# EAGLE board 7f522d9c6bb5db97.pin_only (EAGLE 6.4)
REV: B

Size 25.4 x 25.4 mm. Coordinates in mm from the lower left corner, seen from the top.
Outline: circle at 12.7,12.7 radius 12.7
Copper layers (1*16): Top 0.035mm / dielectric 1.5mm / Bottom 0.035mm
Design rules "adafruit *": minimum track width 8mil, minimum drill 15.5mil, track to track 8mil, track to pad 8mil, pad to pad 8mil, via to via 8mil, smd to smd 8mil, copper to edge 10mil, drill to drill 8mil, minimum pad ring 10mil, minimum via ring 8mil, stop-mask expansion 4mil, vias tented up to drill 20mil, thermal gap 10mil
Net classes: 1 GND: width 0.305 mm; 2 VIN: width 0.305 mm; 3 +3.3: width 0.305 mm
Holes 2.8 mm at 2.54,12.7 22.86,12.7

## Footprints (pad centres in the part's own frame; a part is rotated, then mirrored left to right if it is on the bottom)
0805-NO = smd 1.24 x 1.5: 1 -0.95,0; 2 0.95,0
FIDUCIAL_1MM = smd 1 x 1: 1 0,0
SEWALLI = drill 3.2: P$1 0,0.508
SOT363 = smd 0.5 x 0.5: 1 -0.75,-0.9; 3 0.75,-0.9; 4 0.75,0.9; 6 -0.75,0.9 | smd 0.4 x 0.5: 2 0,-0.9; 5 0,0.9
RESPACK_4X0603 = smd 0.45 x 0.9: 1 -1.3,-0.85; 2 -0.4,-0.85; 3 0.4,-0.85; 4 1.3,-0.85; 5 1.3,0.85; 6 0.4,0.85; 7 -0.4,0.85; 8 -1.3,0.85
SOLDERJUMPER_2WAY_OPEN_NOPASTE = smd 1.168 x 1.6: 1 -1.397,0; 2 0,0; 3 1.397,0
SOT23-5 = smd 0.55 x 1.2: 1 -0.95,-1.3; 2 0,-1.3; 3 0.95,-1.3; 4 0.95,1.3; 5 -0.95,1.3
TSL2561_FN = smd 1.3 x 0.4: ADR -0.8,0; CLK 0.8,-0.65; DATA 0.8,0.65; INT 0.8,0; VDD -0.8,0.65; VSS -0.8,-0.65
JSTPH4 = smd 1 x 4.6: 1 -3,-3.7; 2 -1,-3.7; 3 1,-3.7; 4 3,-3.7 | smd 1.7 x 3.4: NC1 -5.7,1.5; NC2 5.7,1.5

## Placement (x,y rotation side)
C1  10uF  [0805-NO]  11.68,11.85 270 top
C2  10uF  [0805-NO]  6.06,11.98 270 top
FID1  FIDUCIAL_1MM  [FIDUCIAL_1MM]  9.02,19.94 0 top
FID2  FIDUCIAL_1MM  [FIDUCIAL_1MM]  16.38,22.1 0 top
GND_PAD  SEWTAP-ALLIGATOR  [SEWALLI]  4.06,7.62 120 top
Q3  2N7002D  [SOT363]  14.22,11.62 90 top
R1  10K  [RESPACK_4X0603]  17.27,11.81 270 top
SCL_PAD  SEWTAP-ALLIGATOR  [SEWALLI]  4.06,17.78 60 top
SDA_PAD  SEWTAP-ALLIGATOR  [SEWALLI]  21.34,17.78 300 top
SJ1  [SOLDERJUMPER_2WAY_OPEN_NOPASTE]  9.02,8 270 bottom
U2  MIC5225-3.3  [SOT23-5]  8.93,11.64 180 top
U3  TSL2561  [TSL2561_FN]  12.7,6.35 0 top
U$4  [STEMMA_TSL2561_B_FRONT]  0,0 0 top
U$7  [STEMMA_TSL2561_B_BACK]  25.4,0 0 bottom
U$8  [PCBFEAT-REV-040]  5.65,12.51 0 bottom
VIN_PAD  SEWTAP-ALLIGATOR  [SEWALLI]  21.34,7.62 240 top
X1  STEMMA_I2C_RASMT  [JSTPH4]  12.7,20.19 0 top

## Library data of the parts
C1 C2 GND_PAD Q3 R1 SCL_PAD SDA_PAD SJ1 U2 U3 U$8 VIN_PAD X1 = microbuilder
FID1 FID2 = microbuilder; BOM: EXCLUDE
U$4 U$7 = silks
